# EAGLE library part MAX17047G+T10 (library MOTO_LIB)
Fuel Guage
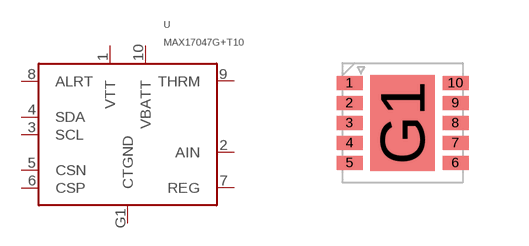
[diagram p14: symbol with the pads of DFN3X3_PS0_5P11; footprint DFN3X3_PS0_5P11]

Designator prefix -

## MAX17047G+T10 (MPN: MAX17047G+T10; SUPPLIER: MAXIM)  [DFN3X3_PS0_5P11]
1  VTT
2  AIN
3  SCL
4  SDA
5  CSN
6  CSP
7  REG
8  ALRT
9  THRM
10  VBATT
G1  CTGND

## Footprint DFN3X3_PS0_5P11 (pad centres in mm)
smd 0.65 x 0.35: 1 -1.325,1; 2 -1.325,0.5; 3 -1.325,0; 4 -1.325,-0.5; 5 -1.325,-1; 6 1.325,-1; 7 1.325,-0.5; 8 1.325,0; 9 1.325,0.5; 10 1.325,1
smd 1.6 x 2.4: G1 0,0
